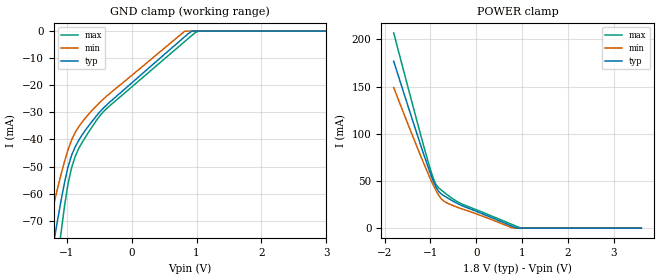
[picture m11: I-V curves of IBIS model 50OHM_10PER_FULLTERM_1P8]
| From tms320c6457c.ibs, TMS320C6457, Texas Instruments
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|   Model Cell 50OHM_10PER_FULLTERM_1P8
|50OHM_10PER_FULLTERM_1P8
[Model]   50OHM_10PER_FULLTERM_1P8
Model_type   Input
Polarity   Non-Inverting
Vinl =  0.8
Vinh =  1
C_comp   1.89p   1.72p   2.18p
[Model Spec]
Vinl   0.8   0.71   0.89
Vinh   1   0.91   1.09
D_overshoot_high 2.34 NA NA
D_overshoot_low -0.54 NA NA
D_overshoot_time 0.56n NA NA
S_overshoot_high 2.2 NA NA
S_overshoot_low -0.4 NA NA
[Receiver Thresholds]
Vth = 0.9V
Vth_min = 0.855V
Vth_max = 0.945V
Vinl_dc = -125mV
Vinh_dc = +125mV
Vinl_ac = -250mV
Vinh_ac = +250mV
Tslew_ac = 5.000ns
Threshold_sensitivity = 0.50
Reference_supply Pullup_ref
[Temperature Range]   25   125   -40
[Voltage Range]   1.8   1.62   1.98
[Pullup reference]   1.8   1.62   1.98
[POWER_clamp]
|   voltage   I(typ)   I(min)   I(max)
-1.8V     177mA      149.1mA    206.9mA
-1.255V   94.38mA    81.75mA    106.6mA
-981.8mV  55.59mA    50.37mA    59.44mA
-927.3mV  48.77mA    44.64mA    51.58mA
-872.7mV  42.93mA    39.34mA    45.82mA
-818.2mV  38.76mA    34.72mA    42.61mA
-709.1mV  34.49mA    28.75mA    38.28mA
-327.3mV  24.2mA     20.72mA    25.99mA
763.6mV   2.439mA    695.1uA    4.262mA
872.7mV   187.6uA    0A         2.048mA
981.8mV   0A         0A         0A
3.6V      0A         0A         0A
[GND_clamp]
|   voltage   I(typ)   I(min)   I(max)
-1.8V     -171.2mA   -131.6mA   -226.7mA
-1.309V   -93.92mA   -75.54mA   -119.5mA
-1.2V     -77.93mA   -63.94mA   -96.64mA
-1.145V   -70.25mA   -58.42mA   -85.54mA
-1.091V   -62.88mA   -53.15mA   -74.81mA
-981.8mV  -50.24mA   -43.86mA   -56.48mA
-927.3mV  -45.91mA   -40.26mA   -50.57mA
-818.2mV  -40.41mA   -35.38mA   -43.42mA
-600mV    -33.02mA   -29.01mA   -34.96mA
818.2mV   -2.072mA   -59.49uA   -3.845mA
1.036V    0A         0A         0A
3.6V      0A         0A         0A
